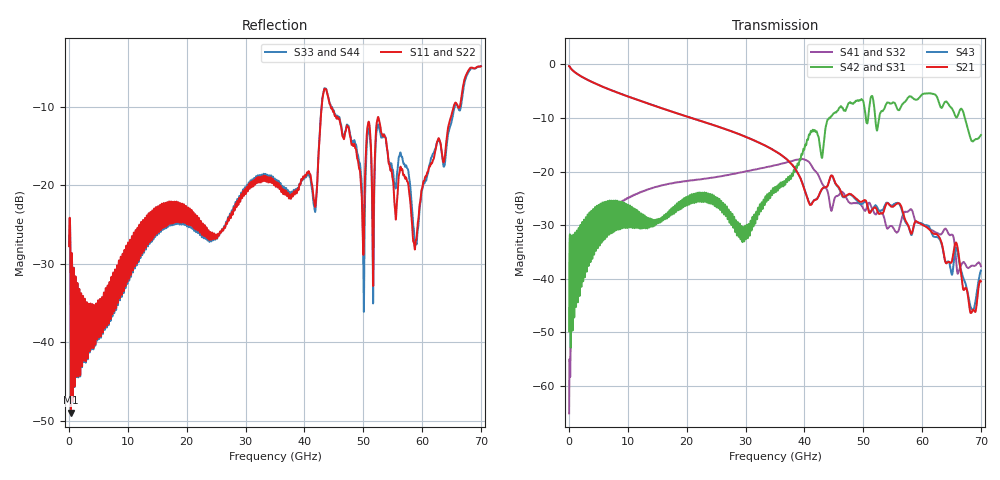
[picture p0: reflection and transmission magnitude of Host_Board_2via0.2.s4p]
! AWR Design Environment (8415) Wed Sep 26 16:40:26 2018
! Document = 'Host PCB'
! nPorts: 4, nXvals: 7001
# HZ S DB R 50
!Freq DBS11 AngS11 DBS12 AngS12 DBS13 AngS13 DBS14 AngS14
!	DBS21 AngS21 DBS22 AngS22 DBS23 AngS23 DBS24 AngS24
!	DBS31 AngS31 DBS32 AngS32 DBS33 AngS33 DBS34 AngS34
!	DBS41 AngS41 DBS42 AngS42 DBS43 AngS43 DBS44 AngS44
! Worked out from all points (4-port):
!   7000 points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, 10 MHz to 70 GHz, reference 50 ohm
!   strongest paths, dB at 10 MHz, 17.51 GHz, 35.01 GHz, 52.51 GHz, 70 GHz:
!     S21: -0.4, -8.8, -16.2, -27.7, -40.5
!     S43: -0.4, -8.8, -16.2, -27.1, -38.4
!     S42: -49.8, -27.8, -23.0, -11.3, -13.2
!     S31: -49.8, -27.8, -23.0, -11.3, -13.2
!     S41: -65.1, -22.2, -18.8, -27.4, -37.6
!     S32: -65.1, -22.2, -18.8, -27.4, -37.6
!   lowest |S11| = -48.9 dB at 310 MHz (marker M1), VSWR 1.01, Z = 50.3 - j0.213 ohm
!   |S11| at or under -10 dB: start of sweep to 42.93 GHz; 44.49 GHz to 65.35 GHz (20.86 GHz wide, 38 % of centre); 66.10657 GHz to 66.40493 GHz (298.4 MHz wide, 0.45 % of centre)
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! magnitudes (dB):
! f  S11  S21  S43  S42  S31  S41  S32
! 10 MHz  -27.7  -0.4  -0.4  -49.8  -49.8  -65.1  -65.1
! 310 MHz  -48.9  -0.8  -0.8  -45.1  -45.1  -49.7  -49.7
! 3.81 GHz  -40.7  -3.3  -3.3  -27.4  -27.4  -30.9  -30.9
! 16.98 GHz  -22.3  -8.6  -8.6  -28.2  -28.2  -22.3  -22.3
! 43.56 GHz  -7.7  -22.9  -22.9  -12.1  -12.1  -23.0  -23.0
! 58.78 GHz  -28.1  -29.5  -29.5  -6.5  -6.5  -29.0  -29.0
! 70 GHz  -4.8  -40.5  -38.4  -13.2  -13.2  -37.6  -37.6
